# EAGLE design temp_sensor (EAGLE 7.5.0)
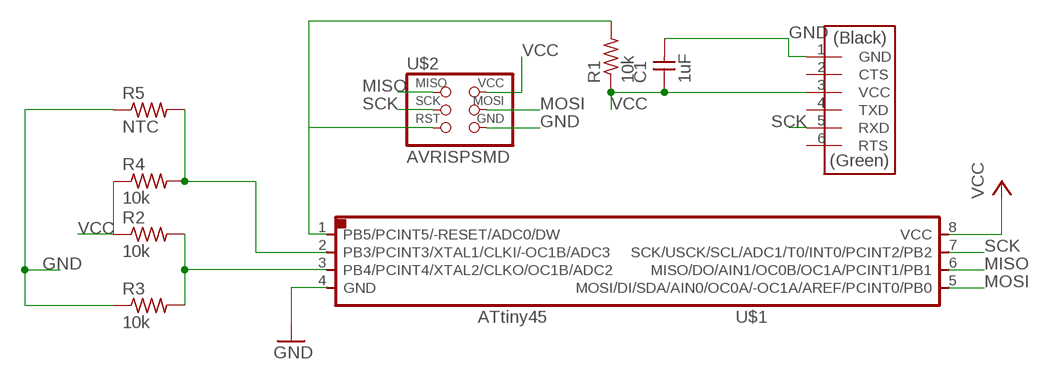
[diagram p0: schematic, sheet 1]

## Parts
C1  1uF  CAP-UNPOLARIZEDFAB  [C1206FAB]
R1  10k  RES-US1206FAB  [R1206FAB]
R2  10k  RES-US1206FAB  [R1206FAB]
R3  10k  RES-US1206FAB  [R1206FAB]
R4  10k  RES-US1206FAB  [R1206FAB]
R5  NTC  RES-US1206FAB  [R1206FAB]
U$1  ATTINY45SI  [SOIC8]
U$2  AVRISPSMD  [2X03SMD]
U$3  FTDI-SMD-HEADER  [1X06SMD]

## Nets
GND: C1.2 R3.1 R5.1 U$1.4(GND) U$2.6(GND) U$3.1(GND)
MISO: U$1.6(MISO/DO/AIN1/OC0B/OC1A/PCINT1/PB1) U$2.1(MISO)
MOSI: U$1.5(MOSI/DI/SDA/AIN0/OC0A/-OC1A/AREF/PCINT0/PB0) U$2.4(MOSI)
N$1: R1.2 U$1.1(PB5/PCINT5/-RESET/ADC0/DW) U$2.5(RST)
N$2: R4.2 R5.2 U$1.2(PB3/PCINT3/XTAL1/CLKI/-OC1B/ADC3)
N$3: R2.2 R3.2 U$1.3(PB4/PCINT4/XTAL2/CLKO/OC1B/ADC2)
SCK: U$1.7(SCK/USCK/SCL/ADC1/T0/INT0/PCINT2/PB2) U$2.3(SCK) U$3.5(RXD)
VCC: C1.1 R1.1 R2.1 R4.1 U$1.8(VCC) U$2.2(VCC) U$3.3(VCC)
Unconnected: U$3.2(CTS) U$3.4(TXD) U$3.6(RTS)

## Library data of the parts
C1 = fab:CAP-UNPOLARIZED
R1-R5 = fab:RES-US: Resistor (US Symbol)
U$1 = fab:ATTINY45
U$2 = fab:AVRISP
U$3 = fab:FTDI-SMD-HEADER

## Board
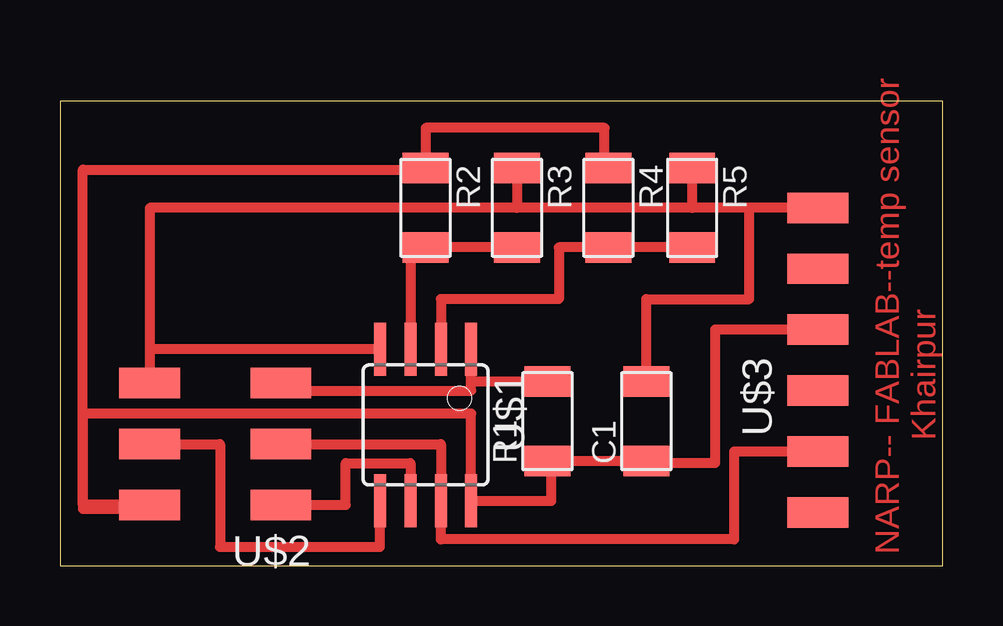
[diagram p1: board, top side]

Size 36.81 x 19.36 mm. Coordinates in mm from the lower left corner, seen from the top.
Outline: 0,0 36.81,0 36.81,19.36 0,19.36 0,0
Copper layers (1*16): Top 0.035mm / dielectric 1.5mm / Bottom 0.035mm
Design rules "default": minimum track width 10mil, minimum drill 24mil, track to track 8mil, track to pad 8mil, pad to pad 8mil, via to via 8mil, smd to smd 8mil, copper to edge 40mil, drill to drill 8mil, minimum pad ring 10mil, minimum via ring 8mil, stop-mask expansion 4mil, vias tented up to drill 0mil, thermal gap 10mil

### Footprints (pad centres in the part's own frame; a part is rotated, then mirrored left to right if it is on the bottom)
C1206FAB = smd 1.27 x 1.905: 1 -1.651,0; 2 1.651,0
R1206FAB = smd 1.27 x 1.905: 1 -1.651,0; 2 1.651,0
SOIC8 = smd 0.5 x 2.2: 1 -1.905,-3.154; 2 -0.645,-3.154; 3 0.625,-3.154; 4 1.895,-3.154; 5 1.905,3.154; 6 0.635,3.154; 7 -0.635,3.154; 8 -1.905,3.154
2X03SMD = smd 2.54 x 1.27: 1 -2.54,2.54; 2 2.92,2.54; 3 -2.54,0; 4 2.92,0; 5 -2.54,-2.54; 6 2.92,-2.54
1X06SMD = smd 2.54 x 1.27: 1 0,6.35; 2 0,3.81; 3 0,1.27; 4 0,-1.27; 5 0,-3.81; 6 0,-6.35

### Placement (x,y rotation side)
C1  24.45,6.03 90 top
R1  20.32,6.03 90 top
R2  15.24,14.92 270 top
R3  19.05,14.92 270 top
R4  22.86,14.92 270 top
R5  26.35,14.92 270 top
U$1  15.24,5.87 180 top
U$2  6.67,5.08 180 top
U$3  31.59,8.57 0 top

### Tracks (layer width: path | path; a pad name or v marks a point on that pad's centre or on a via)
GND
  Top 0.406: U$3.1 28.73,14.92 | 28.73,14.92 26.35,14.92 | R5.1 26.35,14.92 | 26.35,14.92 19.05,14.92 | R3.1 19.05,14.92 | 19.05,14.92 3.75,14.92 3.75,9.03 | 3.75,9.03 U$2.6 | U$1.4 3.75,9.03 | C1.2 24.45,11.11 28.73,11.11 28.73,14.92
MISO
  Top 0.406: U$2.1 11.91,2.54 11.91,4.29 14.61,4.29 U$1.6
MOSI
  Top 0.406: U$2.4 6.67,5.08 6.67,0.79 13.34,0.79 U$1.5
N$1
  Top 0.406: 17.14,7.68 U$1.1 | R1.2 17.14,7.68 | U$2.5 10.16,7.62 10.16,7.3 17.14,7.3 17.14,7.68
N$2
  Top 0.406: R5.2 R4.2 20.8,13.27 20.8,11.11 15.88,11.11 U$1.2
N$3
  Top 0.406: R3.2 R2.2 14.62,13.27 U$1.3
SCK
  Top 0.406: U$3.5 28.1,4.76 28.1,1.11 15.88,1.11 U$1.7 15.88,5.08 U$2.3
VCC
  Top 0.406: U$3.3 27.3,9.84 27.3,4.29 24.45,4.29 C1.1 R1.1 20.48,4.38 20.48,2.7 17.14,2.7 U$1.8 17.14,6.35 0.95,6.35 0.95,2.38 3.75,2.38 U$2.2 0.95,2.54 0.95,16.51 15.24,16.51 R2.1 15.24,18.26 22.7,18.26 22.7,16.57 R4.1

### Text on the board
Top: NARP-- FABLAB--temp sensor / Khairpur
